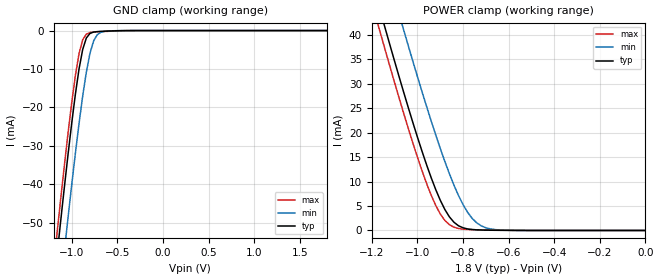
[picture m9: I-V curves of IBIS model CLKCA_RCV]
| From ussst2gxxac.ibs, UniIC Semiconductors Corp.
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|   Model CLKCA_RCV
[Model]  CLKCA_RCV
Model_type Input
Polarity   Non-Inverting
Vinl =   0.70000000V
Vinh =   1.10000000V
C_comp   1.2130pF   1.2100pF   1.2300pF
[Temperature Range]   25.0000   95.0000   0.0
[Voltage Range]   1.8000V   1.7000V   1.9000V
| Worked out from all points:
|   GND clamp passes 1 mA (typ) near -0.81 V on its own axis
|   POWER clamp passes 1 mA (typ) near -0.82 V on its own axis
[GND_clamp]
|Voltage   I(typ)   I(min)   I(max)
-1.8V     -210.2mA   -226.7mA   -204.5mA
-1.16V    -58.1mA    -74.96mA   -52.38mA
-1.12V    -49.19mA   -65.97mA   -43.5mA
-1.08V    -40.49mA   -57.12mA   -34.85mA
-1.04V    -32.04mA   -48.44mA   -26.51mA
-960mV    -16.49mA   -31.85mA   -11.64mA
-920mV    -9.943mA   -24.12mA   -5.959mA
-880mV    -4.898mA   -17mA      -2.383mA
-840mV    -1.924mA   -10.78mA   -923.8uA
-760mV    -381.8uA   -2.67mA    -388.6uA
-640mV    -161.4uA   -198.1uA   -231.6uA
1.8V      42.45pA    124.6pA    90.35pA
[POWER_clamp]
|Voltage   I(typ)   I(min)   I(max)
-1.8V     156.2mA    168.8mA    151.8mA
-1.18V    47.75mA    60.71mA    43.3mA
-1.16V    44.42mA    57.36mA    39.98mA
-1.14V    41.11mA    54.04mA    36.69mA
-1.06V    28.22mA    40.96mA    23.91mA
-940mV    10.82mA    22.44mA    7.238mA
-880mV    4.308mA    14.14mA    2.067mA
-840mV    1.685mA    9.283mA    678.2uA
-800mV    541.2uA    5.283mA    274.7uA
-760mV    193.2uA    2.472mA    165.1uA
-680mV    54.36uA    319.1uA    87.85uA
0V        42.45pA    73.31pA    95.52pA
